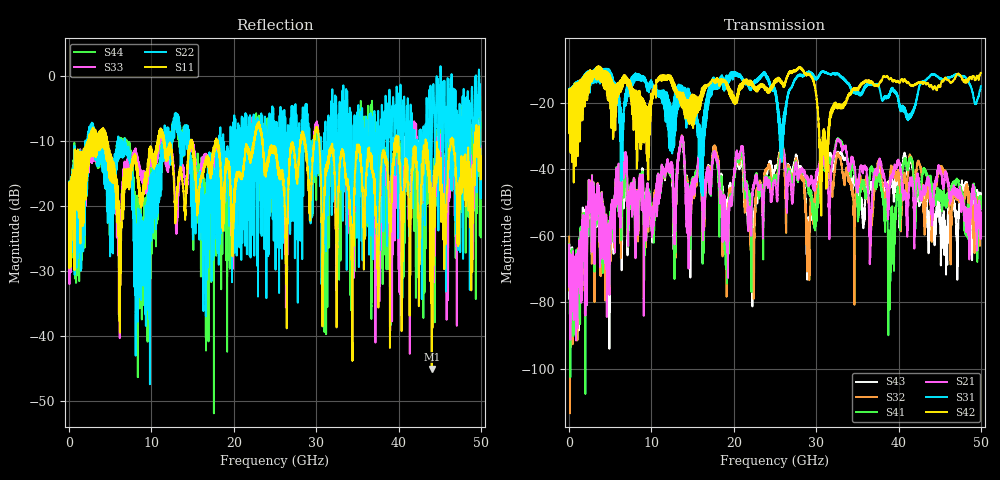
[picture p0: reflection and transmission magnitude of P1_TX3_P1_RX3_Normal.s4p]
!Keysight Technologies,N5225B,MY57041031,A.13.20.10
!Date: Friday, May 31, 2019 11:17:18
!Correction: S11(Full 4 Port(1,2,3,4))
!S12(Full 4 Port(1,2,3,4))
!S13(Full 4 Port(1,2,3,4))
!S14(Full 4 Port(1,2,3,4))
!S21(Full 4 Port(1,2,3,4))
!S22(Full 4 Port(1,2,3,4))
!S23(Full 4 Port(1,2,3,4))
!S24(Full 4 Port(1,2,3,4))
!S31(Full 4 Port(1,2,3,4))
!S32(Full 4 Port(1,2,3,4))
!S33(Full 4 Port(1,2,3,4))
!S34(Full 4 Port(1,2,3,4))
!S41(Full 4 Port(1,2,3,4))
!S42(Full 4 Port(1,2,3,4))
!S43(Full 4 Port(1,2,3,4))
!S44(Full 4 Port(1,2,3,4))
!S4P File: Measurements: <S11,S12,S13,S14>,
!<S21,S22,S23,S24>,
!<S31,S32,S33,S34>,
!<S41,S42,S43,S44>:
# Hz S  dB  R 50.0
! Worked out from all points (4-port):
!   5000 points, 10 MHz to 50 GHz, reference 50 ohm
!   strongest paths, dB at 10 MHz, 12.51 GHz, 25.01 GHz, 37.51 GHz, 50 GHz:
!     S42: -19.7, -14.4, -13.3, -14.9, -10.9
!     S31: -19.4, -27.1, -15.8, -14.5, -15.0
!     S21: -62.7, -40.9, -43.3, -39.6, -59.1
!     S41: -62.5, -42.0, -41.7, -42.9, -49.5
!     S32: -60.2, -42.0, -42.2, -38.1, -53.2
!     S43: -63.7, -43.3, -39.4, -40.9, -49.0
!   lowest |S11| = -45.1 dB at 44.03 GHz (marker M1), VSWR 1.01, Z = 50.1 + j0.552 ohm
!   |S11| at or under -10 dB: 4.66 GHz to 10.77 GHz (6.107 GHz wide, 79.2 % of centre); 23.49 GHz to 28.08 GHz (4.586 GHz wide, 17.8 % of centre); 30.37 GHz to 39.62 GHz (9.241 GHz wide, 26.4 % of centre)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
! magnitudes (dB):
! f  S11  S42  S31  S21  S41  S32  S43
! 10 MHz  -19.4  -19.7  -19.4  -62.7  -62.5  -60.2  -63.7
! 13.64 GHz  -15.0  -20.8  -14.8  -30.6  -30.8  -30.5  -31.0
! 22.26 GHz  -11.4  -14.4  -15.1  -47.9  -47.4  -60.0  -81.2
! 25.76 GHz  -15.0  -13.3  -27.2  -35.5  -34.8  -34.4  -33.4
! 29.01 GHz  -13.9  -11.3  -11.1  -43.2  -45.6  -62.6  -58.2
! 44.03 GHz  -45.1  -15.0  -11.4  -53.8  -44.9  -61.5  -55.1
! 50 GHz  -12.3  -10.9  -15.0  -59.1  -49.5  -53.2  -49.0
